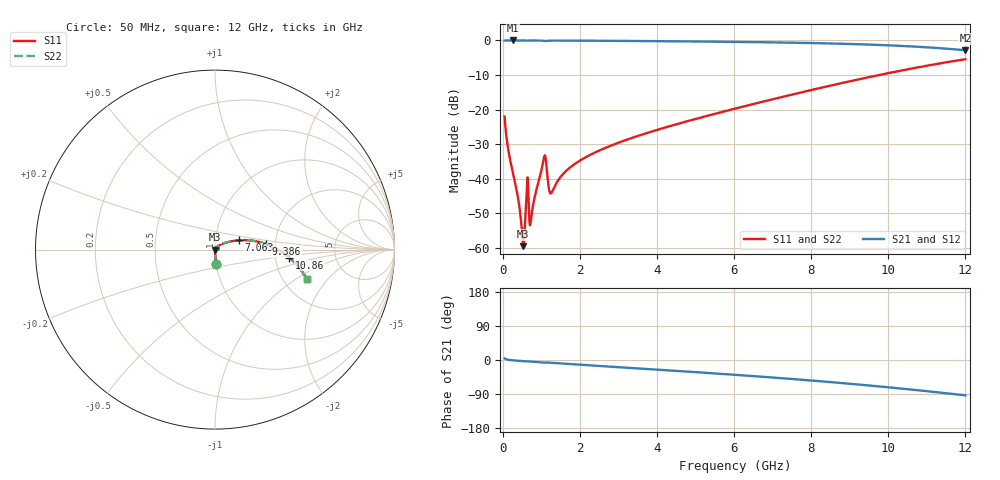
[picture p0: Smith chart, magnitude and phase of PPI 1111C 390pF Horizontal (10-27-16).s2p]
# MHz S MA R 50
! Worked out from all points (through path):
!   1601 points, 50 MHz to 12 GHz, reference 50 ohm
!   highest |S21| = 0.00 dB at 266.6 MHz (marker M1); lowest = -2.8 dB at 12 GHz (marker M2)
!   group delay of S21, straight-line fit = 21 ps
!   lowest |S11| = -59.5 dB at 535.5 MHz (marker M3), VSWR 1.00, Z = 50.1 - j0.024 ohm
!   |S11| at or under -10 dB: start of sweep to 9.766 GHz
!   |S22| runs from -59.5 to -5.4 dB; largest |S21 - S12| = 0
!   S11 on the Smith chart (normalised r, x): 50 MHz: 1.00, -0.16; 7.063 GHz: 1.30, +0.14; 9.386 GHz: 1.79, +0.12; 10.86 GHz: 2.39, -0.26; 12 GHz: 2.68, -1.21
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50  0.07904 -84.8  0.9956 4.2  0.9956 4.2  0.07904 -84.8
266.5938  0.01203 -88.7  0.9995 -0.9  0.9995 -0.9  0.01203 -88.7
401.0312  0.005147 -84.9  0.9993 -2.0  0.9993 -2.0  0.005147 -84.9
498.125  0.001781 -63.1  0.9991 -2.8  0.9991 -2.8  0.001781 -63.1
535.4688  0.001055 -13.1  0.9989 -3.1  0.9989 -3.1  0.001055 -13.1
565.3438  0.001636 36.7  0.9987 -3.3  0.9987 -3.3  0.001636 36.7
625.0938  0.006614 48.1  0.9959 -3.9  0.9959 -3.9  0.006614 48.1
744.5938  0.002842 46.1  0.9981 -4.4  0.9981 -4.4  0.002842 46.1
1065.75  0.01971 42.5  0.987 -7.0  0.987 -7.0  0.01971 42.5
1110.562  0.02043 8.0  0.9802 -6.7  0.9802 -6.7  0.02043 8.0
1207.656  0.00672 3.1  0.9933 -7.0  0.9933 -7.0  0.00672 3.1
1259.938  0.006194 27.6  0.9948 -7.5  0.9948 -7.5  0.006194 27.6
1588.562  0.01204 56.0  0.9949 -9.8  0.9949 -9.8  0.01204 56.0
2044.156  0.01886 54.5  0.9924 -12.8  0.9924 -12.8  0.01886 54.5
4038.312  0.05145 38.3  0.9761 -25.6  0.9761 -25.6  0.05145 38.3
6025  0.1031 26.7  0.9529 -39.1  0.9529 -39.1  0.1031 26.7
7063.156  0.1437 21.2  0.9366 -46.7  0.9366 -46.7  0.1437 21.2
8019.156  0.1925 15.7  0.9169 -54.2  0.9169 -54.2  0.1925 15.7
9385.938  0.2853 6.3  0.8759 -66.2  0.8759 -66.2  0.2853 6.3
10013.31  0.3376 1.3  0.8496 -72.1  0.8496 -72.1  0.3376 1.3
10857.28  0.4166 -6.2  0.8043 -80.7  0.8043 -80.7  0.4166 -6.2
12000  0.5348 -17.6  0.7221 -93.2  0.7221 -93.2  0.5348 -17.6
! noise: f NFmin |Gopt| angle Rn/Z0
50  0.0007724  0.9331  0.3001  0.002571
1372  0.007521  0.8231  7.908  0.008879
2701  0.01711  0.8467  15.48  0.02329
4031  0.02896  0.866  22.9  0.04462
5360  0.04156  0.8782  30.1  0.06883
6682  0.05465  0.8876  37.02  0.09501
8012  0.06873  0.8962  43.69  0.1246
9341  0.08442  0.9049  50.06  0.16
1.067e+04  0.1028  0.9143  56.11  0.2061
1.2e+04  0.1257  0.9244  61.85  0.2713
